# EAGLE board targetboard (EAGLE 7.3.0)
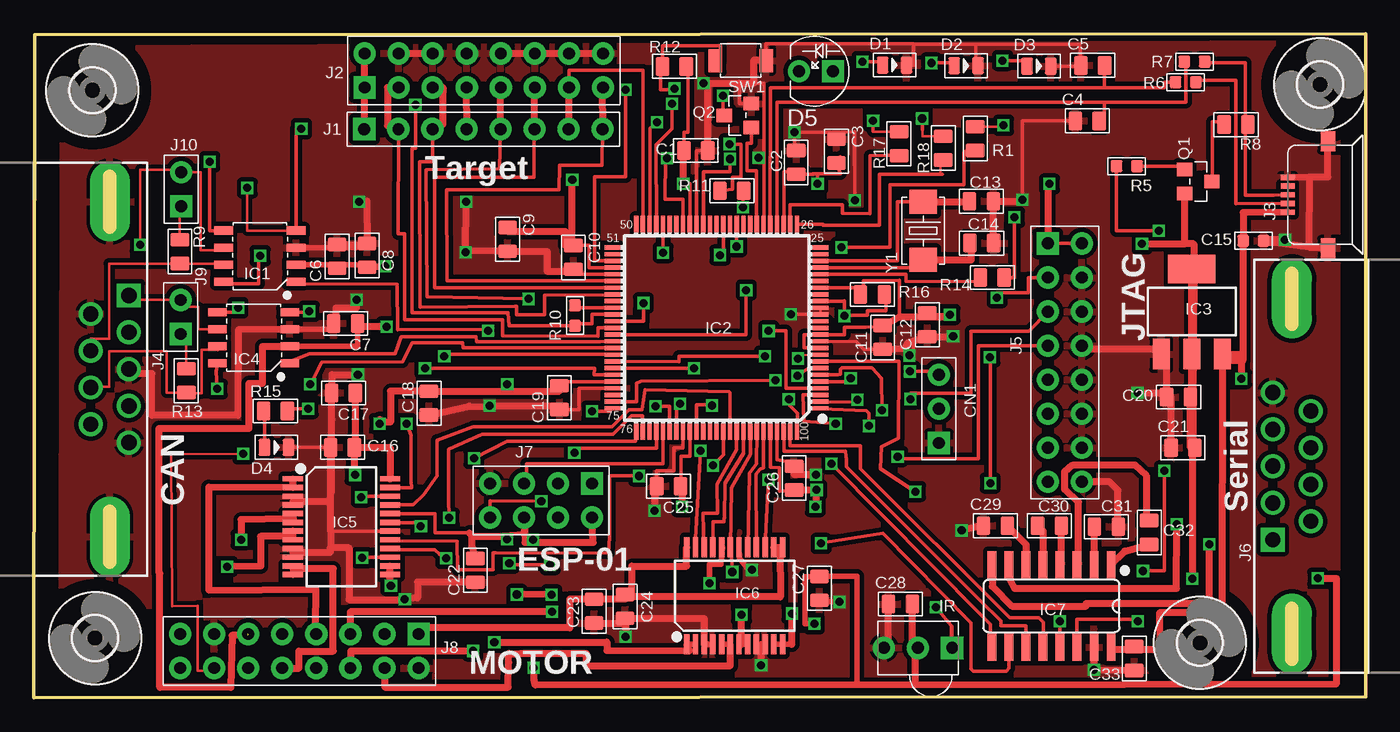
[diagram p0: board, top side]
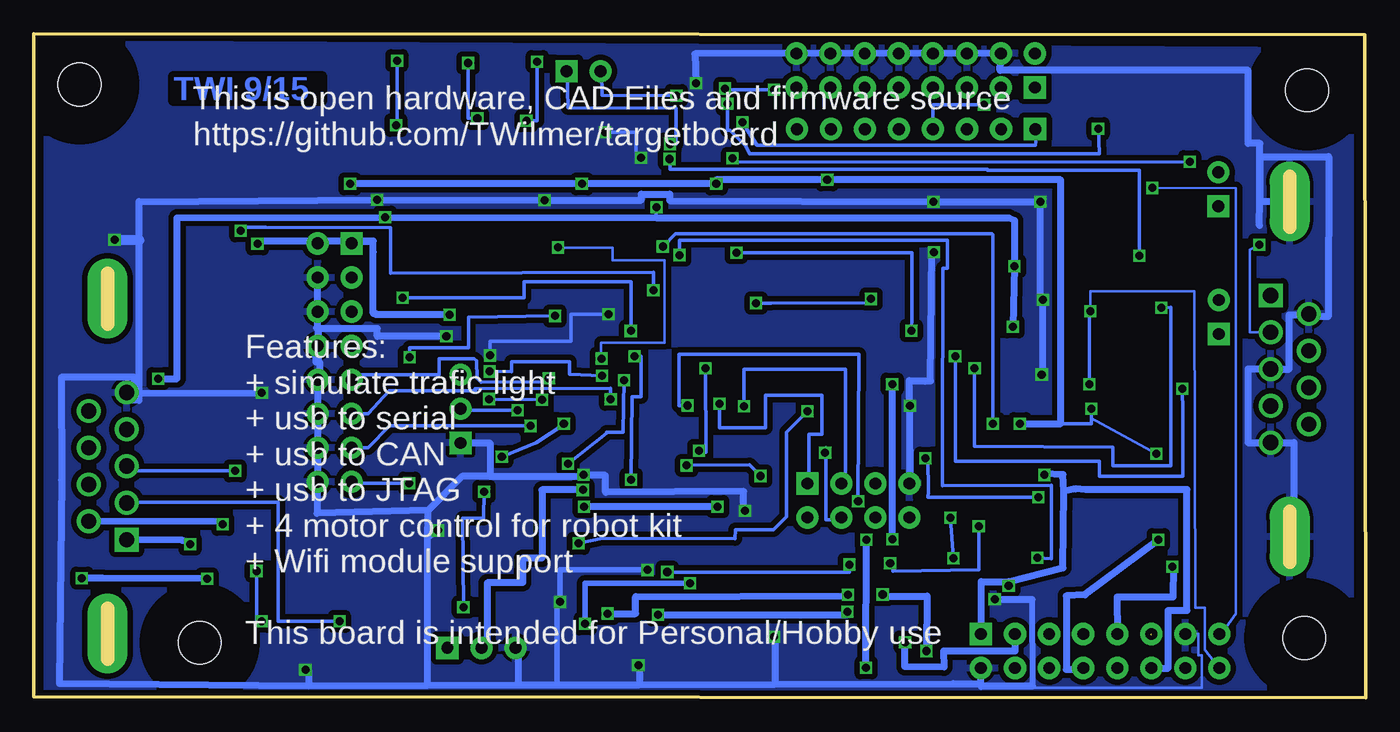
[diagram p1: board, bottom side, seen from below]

Size 99.44 x 49.57 mm. Coordinates in mm from the lower left corner, seen from the top.
Outline: 0,0 99.44,0.08 99.44,49.57 0.1,49.47 0,0
Copper layers (1*16): Top 0.035mm / dielectric 1.5mm / Bottom 0.035mm
Design rules "SeeedStudio_2layer_DRU_no_angle_20140221": minimum track width 7mil, minimum drill 12mil, track to track 7mil, track to pad 7mil, pad to pad 7mil, via to via 7mil, smd to smd 0mil, copper to edge 10mil, drill to drill 10mil, minimum pad ring 10mil, minimum via ring 6mil, stop-mask expansion 2mil, vias tented up to drill 100mil, thermal gap 10mil

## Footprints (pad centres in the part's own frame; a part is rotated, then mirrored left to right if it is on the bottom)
C0805 = smd 1.397 x 1.016: 1 0,0.889; 2 0,-0.889
C0603 = smd 0.889 x 0.889: 1 0,0.762; 2 0,-0.762
H3-2.54 = drill 0.889 pad 1.651 square: 1 0,2.54 | drill 0.889 pad 1.651: 2 0,0; 3 0,-2.54
LED-0805 = smd 0.889 x 1.27: + -0.889,0; - 0.889,0
LED2-2.54-D5.0MM = drill 0.889 pad 1.651 square: + -1.27,0 | drill 0.889 pad 1.651: - 1.27,0
3,2 = hole 3.2: 0,0
SOIC8-1.27-5X4MM = smd 0.6 x 1.4: 1 -1.905,-2.7; 2 -0.635,-2.7; 3 0.635,-2.7; 4 1.905,-2.7; 5 1.905,2.7; 6 0.635,2.7; 7 -0.635,2.7; 8 -1.905,2.7
LQFP100-0.5-13.8X13.8MM = smd 1.2 x 0.32: 1 -7.75,6; 2 -7.75,5.5; 3 -7.75,5; 4 -7.75,4.5; 5 -7.75,4; 6 -7.75,3.5; 7 -7.75,3; 8 -7.75,2.5; 9 -7.75,2; 10 -7.75,1.5; 11 -7.75,1; 12 -7.75,0.5; 13 -7.75,0; 14 -7.75,-0.5; 15 -7.75,-1; 16 -7.75,-1.5; 17 -7.75,-2; 18 -7.75,-2.5; 19 -7.75,-3; 20 -7.75,-3.5; 21 -7.75,-4; 22 -7.75,-4.5; 23 -7.75,-5; 24 -7.75,-5.5; 25 -7.75,-6; 51 7.75,-6; 52 7.75,-5.5; 53 7.75,-5; 54 7.75,-4.5; 55 7.75,-4; 56 7.75,-3.5; 57 7.75,-3; 58 7.75,-2.5; 59 7.75,-2; 60 7.75,-1.5; 61 7.75,-1; 62 7.75,-0.5; 63 7.75,0; 64 7.75,0.5; 65 7.75,1; 66 7.75,1.5; 67 7.75,2; 68 7.75,2.5; 69 7.75,3; 70 7.75,3.5; 71 7.75,4; 72 7.75,4.5; 73 7.75,5; 74 7.75,5.5; 75 7.75,6 | smd 0.32 x 1.2: 26 -6,-7.75; 27 -5.5,-7.75; 28 -5,-7.75; 29 -4.5,-7.75; 30 -4,-7.75; 31 -3.5,-7.75; 32 -3,-7.75; 33 -2.5,-7.75; 34 -2,-7.75; 35 -1.5,-7.75; 36 -1,-7.75; 37 -0.5,-7.75; 38 0,-7.75; 39 0.5,-7.75; 40 1,-7.75; 41 1.5,-7.75; 42 2,-7.75; 43 2.5,-7.75; 44 3,-7.75; 45 3.5,-7.75; 46 4,-7.75; 47 4.5,-7.75; 48 5,-7.75; 49 5.5,-7.75; 50 6,-7.75; 76 6,7.75; 77 5.5,7.75; 78 5,7.75; 79 4.5,7.75; 80 4,7.75; 81 3.5,7.75; 82 3,7.75; 83 2.5,7.75; 84 2,7.75; 85 1.5,7.75; 86 1,7.75; 87 0.5,7.75; 88 0,7.75; 89 -0.5,7.75; 90 -1,7.75; 91 -1.5,7.75; 92 -2,7.75; 93 -2.5,7.75; 94 -3,7.75; 95 -3.5,7.75; 96 -4,7.75; 97 -4.5,7.75; 98 -5,7.75; 99 -5.5,7.75; 100 -6,7.75
SOT-223 = smd 1.27 x 2.286: 1 -2.286,-3.175; 2 0,-3.175; 3 2.286,-3.175 | smd 3.556 x 2.159: TER 0,3.175
SSOP24-0.65-8.9X5.3MM = smd 0.4 x 1.5: 1 -3.575,-3.625; 2 -2.925,-3.625; 3 -2.275,-3.625; 4 -1.625,-3.625; 5 -0.975,-3.625; 6 -0.325,-3.625; 7 0.325,-3.625; 8 0.975,-3.625; 9 1.625,-3.625; 10 2.275,-3.625; 11 2.925,-3.625; 12 3.575,-3.625; 13 3.575,3.625; 14 2.925,3.625; 15 2.275,3.625; 16 1.625,3.625; 17 0.975,3.625; 18 0.325,3.625; 19 -0.325,3.625; 20 -0.975,3.625; 21 -1.625,3.625; 22 -2.275,3.625; 23 -2.925,3.625; 24 -3.575,3.625
SOIC16-1.27-10X3.9MM = smd 0.66 x 2.032: 1 -4.445,-3.073; 2 -3.175,-3.073; 3 -1.905,-3.073; 4 -0.635,-3.073; 5 0.635,-3.073; 6 1.905,-3.073; 7 3.175,-3.073; 8 4.445,-3.073; 9 4.445,3.073; 10 3.175,3.073; 11 1.905,3.073; 12 0.635,3.073; 13 -0.635,3.073; 14 -1.905,3.073; 15 -3.175,3.073; 16 -4.445,3.073
SNR3-2.54-6.95X6.0X5.6MM = drill 0.889 pad 1.651 square: 1 0,2.54 | drill 0.889 pad 1.651: 2 0,0; 3 0,-2.54
H8-2.54 = drill 0.889 pad 1.651 square: 1 0,8.89 | drill 0.889 pad 1.651: 2 0,6.35; 3 0,3.81; 4 0,1.27; 5 0,-1.27; 6 0,-3.81; 7 0,-6.35; 8 0,-8.89
H2X8-2.54 = drill 0.889 pad 1.651 square: 1 -1.27,8.89 | drill 0.889 pad 1.651: 2 -1.27,6.35; 3 -1.27,3.81; 4 -1.27,1.27; 5 -1.27,-1.27; 6 -1.27,-3.81; 7 -1.27,-6.35; 8 -1.27,-8.89; 9 1.27,-8.89; 10 1.27,-6.35; 11 1.27,-3.81; 12 1.27,-1.27; 13 1.27,1.27; 14 1.27,3.81; 15 1.27,6.35; 16 1.27,8.89
MICRO-USB5+2P-SMD-0.65 = smd 0.4 x 1.05: 1 -1.3,0; 2 -0.65,0; 3 0,0; 4 0.65,0; 5 1.3,0 | smd 1.5 x 1.1: 6 4,-3; 7 -4,-3
DSUB9+2P-2.77-90D-MALE = drill 1.143 pad 1.778 square: 1 -5.486,1.422 | drill 1.143 pad 1.778: 2 -2.743,1.422; 3 0,1.422; 4 2.743,1.422; 5 5.486,1.422; 6 -4.115,-1.422; 7 -1.372,-1.422; 8 1.372,-1.422; 9 4.115,-1.422 | drill 1 pad 3 long: G1 12.497,0; G2 -12.497,0
H2X4-2.54 = drill 0.889 pad 1.651 square: 1 -1.27,3.81 | drill 0.889 pad 1.651: 2 -1.27,1.27; 3 -1.27,-1.27; 4 -1.27,-3.81; 5 1.27,-3.81; 6 1.27,-1.27; 7 1.27,1.27; 8 1.27,3.81
H2-2.54 = drill 0.889 pad 1.651 square: 1 0,1.27 | drill 0.889 pad 1.651: 2 0,-1.27
SOT-23 = smd 1.016 x 1.143: 1 -0.889,-1.016; 2 0.889,-1.016; 3 0,1.016
R0805 = smd 1.397 x 1.016: 1 0,0.889; 2 0,-0.889
R0603 = smd 0.889 x 0.889: 1 0,0.762; 2 0,-0.762
SW2-2.6-3.0X2.5X1.2+0.4MM = smd 1 x 1.7: 1 -1.9,0; 2 1.9,0
X2-SMD-5.0X3.2X1.3MM = smd 1.778 x 2.032: 1 -2.159,0; 2 2.159,0

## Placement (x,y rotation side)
C1  100nf  [C0805]  49.43,40.84 270 top
C2  100nf  [C0805]  56.92,39.95 0 top
C3  10uf  [C0805]  59.92,40.79 0 top
C4  18pf  [C0805]  78.64,43.05 90 top
C5  18pf  [C0805]  79.04,47.19 90 top
C6  1uf  [C0805]  22.66,32.94 180 top
C7  100nf  [C0805]  23.29,27.94 270 top
C8  100nf  [C0805]  24.89,33.02 180 top
C9  100nf  [C0805]  35.38,34.21 0 top
C10  100nf  [C0805]  40.28,32.87 0 top
C11  100nf  [C0805]  63.37,26.9 180 top
C12  100nf  [C0805]  66.7,27.84 180 top
C13  18pf  [C0805]  70.74,37.06 270 top
C14  18pf  [C0805]  70.76,33.93 270 top
C15  10uf  [C0603]  91.03,34.11 270 top
C16  10uf  [C0805]  23.06,18.69 90 top
C17  100nf  [C0805]  23.14,22.76 270 top
C18  10uf  [C0805]  29.51,22 180 top
C19  100nf  [C0805]  39.24,22.4 180 top
C20  100nf  [C0805]  85.45,22.45 90 top
C21  10uf  [C0805]  85.78,18.67 90 top
C22  100nf  [C0805]  32.97,9.53 180 top
C23  100nf  [C0805]  41.83,6.48 0 top
C24  10uf  [C0805]  44.15,6.83 180 top
C25  100nf  [C0805]  47.4,15.8 270 top
C26  100nf  [C0805]  56.77,16.41 180 top
C27  100nf  [C0805]  58.65,8.18 180 top
C28  10uf  [C0805]  64.69,7.01 90 top
C29  1uf  [C0805]  71.78,12.85 90 top
C30  1uf  [C0805]  75.82,12.85 90 top
C31  1uf  [C0805]  80.06,12.78 90 top
C32  1uf  [C0805]  83.26,12.34 180 top
C33  100nf  [C0805]  82.14,2.95 180 top
CN1  DIP-BLACK-MALE-HEADER-VERT(3P-2.54)  [H3-2.54]  67.56,21.56 180 top
D1  SMD-LED-CLEAR-GREEN(0805)  [LED-0805]  64.26,47.22 0 top
D2  SMD-LED-CLEAR-YELLOW(0805)  [LED-0805]  69.6,47.17 0 top
D3  SMD-LED-CLEAR-RED(0805)  [LED-0805]  75.03,47.14 0 top
D4  SMD-LED-CLEAR-RED(0805)  [LED-0805]  18.14,18.69 0 top
D5  IR 940NM  [LED2-2.54-D5.0MM]  58.39,46.76 180 top
H1  MOUNT-HOLE3.2  [3,2]  4.39,45.34 0 top
H2  MOUNT-HOLE3.2  [3,2]  96.01,45.77 0 top
H3  MOUNT-HOLE3.2  [3,2]  4.6,4.47 0 top
H4  MOUNT-HOLE3.2  [3,2]  87.05,4.11 0 top
IC1  MCP2551  [SOIC8-1.27-5X4MM]  16.89,32.97 90 top
IC2  LPC1768 or LPC1768  [LQFP100-0.5-13.8X13.8MM]  50.98,27.61 180 top
IC3  PMIC-CJT1117-3.3(SOT223)  [SOT-223]  86.44,28.83 0 top
IC4  MCP2551  [SOIC8-1.27-5X4MM]  16.43,26.87 90 top
IC5  TB6612FNG  [SSOP24-0.65-8.9X5.3MM]  22.99,12.78 270 top
IC6  TB6612FNG  [SSOP24-0.65-8.9X5.3MM]  52.32,7.62 0 top
IC7  MAX232D  [SOIC16-1.27-10X3.9MM]  75.97,6.86 180 top
IR  TSOP2238  [SNR3-2.54-6.95X6.0X5.6MM]  66.01,3.73 270 top
J1  DIP-BLACK-MALE-HEADER-VERT(8P-2.54)  [H8-2.54]  33.58,42.44 90 top
J2  2x8p-2.54  [H2X8-2.54]  33.6,46.81 90 top
J3  USB  [MICRO-USB5+2P-SMD-0.65]  93.6,37.54 90 top
J4  CAN  [DSUB9+2P-2.77-90D-MALE]  5.69,24.54 270 top
J5  2x8p-2.54  [H2X8-2.54]  76.96,25.02 0 top
J6  Serial  [DSUB9+2P-2.77-90D-MALE]  93.9,17.3 90 top
J7  2X4P-2.54  [H2X4-2.54]  37.87,14.73 270 top
J8  2x8p-2.54  [H2X8-2.54]  19.84,3.51 270 top
J9  CAN2  [H2-2.54]  10.97,28.42 180 top
J10  CAN1  [H2-2.54]  11.02,37.95 180 top
Q1  PNP-24V  [SOT-23]  86.92,38.53 270 top
Q2  NMOSFET  [SOT-23]  52.55,43.46 90 top
R1  390R  [R0805]  70.28,41.73 180 top
R5  51R  [R0603]  81.58,39.67 90 top
R6  33.2R  [R0603]  85.98,45.95 90 top
R7  33.2R  [R0603]  86.64,47.47 90 top
R8  1.5K  [R0805]  89.74,42.77 270 top
R9  120R  [R0805]  10.92,33.3 0 top
R10  330R  [R0603]  40.41,28.52 0 top
R11  100R  [R0805]  52.12,37.85 90 top
R12  1.5K  [R0805]  47.83,47.12 90 top
R13  120R  [R0805]  11.4,23.67 0 top
R14  1.5K  [R0805]  71.55,31.37 270 top
R15  100R  [R0805]  18.06,21.41 90 top
R16  2K  [R0805]  62.61,30.1 270 top
R17  390R  [R0805]  64.59,41.35 180 top
R18  390R  [R0805]  67.89,41.02 180 top
SW1  SW  [SW2-2.6-3.0X2.5X1.2+0.4MM]  52.78,47.55 180 top
Y1  12MHZ  [X2-SMD-5.0X3.2X1.3MM]  66.4,34.85 90 top

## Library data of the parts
C1 C2 C7-C12 C17 C19 C20 C22 C23 C25-C27 C33 = Seeed-OPL-Capacitor; MPN: CC0805KRX7R9BB104
C3 C16 C18 C21 C24 C28 = Seeed-OPL-Capacitor; MPN: CC0805KKX5R8BB106
C4 C5 C13 C14 = Seeed-OPL-Capacitor
C6 C29-C32 = Seeed-OPL-Capacitor; MPN: CC0805KKX7R8BB105
C15 = Seeed-OPL-Capacitor; MPN: CC0603KRX5R6BB106
CN1 J4 J6 J7 = Seeed-OPL-Connector
D1 = Seeed-OPL-Diode; MPN: 17-215SYGC/S530-E2/TR8
D2 = Seeed-OPL-Diode; MPN: 17-215UYC/S530-A3/TR8
D3 D4 = Seeed-OPL-Diode; MPN: 17-215SURC/S530-A2/TR8
D5 = Seeed-OPL-Diode; MPN: IR523B-W60W1
H1-H4 = holes
IC1 IC4 = Seeed-OPL-ic; MPN: MCP2551-I/SN
IC2 = Seeed-OPL-ic; MPN: LPC1768FBD100
IC3 = Seeed-OPL-ic; MPN: CJT1117-3.3
IC5 IC6 = Seeed-OPL-ic; MPN: TB6612FNG-O/C8/EL
IC7 = Seeed-OPL-ic; MPN: MAX232D
IR = Seeed-OPL-sensor
J1 = Seeed-OPL-Connector; MPN: P125-1108A1BS116A1
J2 J5 J8 = Seeed-OPL-Connector; MPN: P125-1216A0AS116A1
J3 = Seeed-OPL-Connector; MPN: ST-USB-001L
J9 J10 = Seeed-OPL-Connector; MPN: P125-1102A0BS116A3
Q1 = Seeed-OPL-Transistor; MPN: S8550
Q2 = Seeed-OPL-Transistor; MPN: 2N7002,215
R1 R17 R18 = Seeed-OPL-Resistor; MPN: RC0805JR-07390RL
R5 = Seeed-OPL-Resistor; MPN: RC0603FR-0751RL
R6 R7 = Seeed-OPL-Resistor; MPN: RC0603FR-0733R2L
R8 R12 R14 = Seeed-OPL-Resistor; MPN: RC0805FR-071K5L
R9 R13 = Seeed-OPL-Resistor; MPN: RC0805JR-07120RL
R10 = Seeed-OPL-Resistor; MPN: RC0603FR-07330RL
R11 R15 = Seeed-OPL-Resistor; MPN: RC0805JR-07100RL
R16 = Seeed-OPL-Resistor; MPN: RC0805JR-072KL
SW1 = Seeed-OPL-Switch
Y1 = Seeed-OPL-crystal-osctllator; MPN: 5032/2P

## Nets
+12V: C16.2 C17.1 C23.1 C24.2 IC5.13 IC5.14 IC5.24 IC6.13 IC6.14 IC6.24 J8.1 J8.11
CAN1_H: IC1.7 J4.7 R9.2
CAN1_L: IC1.6 J4.2 J10.2
CAN1_REF: IC1.5 IC2.43
CAN1_RS: IC1.8 IC2.40
CAN1_RX: IC1.4 IC2.47 J8.8
CAN1_TX: IC1.1 IC2.46
CAN2_H: IC4.7 J4.8 R13.2
CAN2_L: IC4.6 J4.1 J9.2
CAN2_REF: IC2.70 IC4.5
CAN2_RS: IC2.67 IC4.8
CAN2_RX: IC2.66 IC4.4 J8.9
CAN2_TX: IC2.65 IC4.1
CM1A: IC2.91 IC6.22
CM1B: IC2.92 IC6.21
CM2A: IC2.94 IC6.17
CM2B: IC2.95 IC6.16
CM3A: IC2.76 IC5.22
CM3B: IC2.90 IC5.21
CM4A: IC2.89 IC5.17
CM4B: IC2.77 IC5.16
DM: J3.2 R6.2
DP: J3.3 R7.2 R8.1
EDM: C5.2 IC2.30 R6.1
EDP: C4.2 IC2.29 R7.1
ESP_0: IC2.81 J7.2
ESP_2: IC2.80 J7.3
ESP_RST: IC2.79 J7.7
GND: C1.1 C2.1 C3.1 C4.1 C5.1 C6.2 C7.2 C8.2 C9.2 C10.2 C11.1 C12.1 C13.1 C14.1 C15.1 C16.1 C17.2 C18.1 C19.1 C20.1 C21.1 C22.1 C23.2 C24.1 C25.2 C26.2 C27.1 C28.1 C29.1 C31.2 C33.1 CN1.1 D1.- D2.- D3.- D4.- IC1.3 IC2.11 IC2.15 IC2.16 IC2.31 IC2.41 IC2.55 IC2.72 IC2.83 IC2.97 IC3.1 IC4.3 IC5.3 IC5.4 IC5.9 IC5.10 IC5.18 IC6.3 IC6.4 IC6.9 IC6.10 IC6.18 IC7.15 IR.3 J2.9 J2.10 J2.11 J2.12 J2.13 J2.14 J2.15 J3.5 J3.6 J3.7 J4.3 J4.5 J4.6 J4.G1 J4.G2 J5.9 J5.10 J5.11 J5.12 J5.13 J5.14 J5.15 J6.5 J7.4 J8.7 J8.16 Q2.2 SW1.1
IR_IN: IC2.8 IR.1
IR_SEND: IC2.32 Q2.1
LED1: IC2.9 R1.1
LED2: IC2.27 R17.1
LED3: IC2.26 R18.1
M1A: IC6.1 IC6.2 J8.2
M1B: IC6.5 IC6.6 J8.15
M2A: IC6.7 IC6.8 J8.3
M2B: IC6.11 IC6.12 J8.14
M3A: IC5.1 IC5.2 J8.4
M3B: IC5.5 IC5.6 J8.13
M4A: IC5.7 IC5.8 J8.5
M4B: IC5.11 IC5.12 J8.12
N$1: IC2.48 J1.1 J2.1 J2.16
N$2: IC2.53 R12.1 SW1.2
N$3: D2.+ R18.2
N$4: D1.+ R17.2
N$5: D3.+ R1.2
N$6: C14.2 IC2.22 Y1.1
N$7: Q1.3 R8.2
N$8: C13.2 IC2.23 Y1.2
N$9: Q1.1 R5.2
N$10: IC2.21 R14.2
N$11: J10.1 R9.1
N$13: J9.1 R13.1
N$14: D5.+ R11.1
N$15: C30.2 IC7.4
N$16: C30.1 IC7.5
N$17: C32.1 IC7.1
N$18: C32.2 IC7.3
N$19: C29.2 IC7.6
N$20: C31.1 IC7.2
N$21: D5.- Q2.3
N$22: IC2.60 R10.1
N$24: D4.+ R15.1
NTRST: IC2.4 J5.2
P2_9: IC2.64 R5.1
PWM1: IC2.69 IC6.23
PWM2: IC2.68 IC6.15
PWM3: IC2.35 IC5.23
PWM4: IC2.37 IC5.15
RST: IC2.17 J5.8 R16.1
RTCK: IC2.100 J5.6
RX3: CN1.2 IC2.6
RX_TO_TX: IC2.85 J7.5
RXD0: IC2.99 IC7.12
RXD1: IC2.74 IC7.9
SER1_RX: IC7.13 J6.2
SER1_TX: IC7.14 J6.3
SER2_RX: IC7.8 J6.1
SER2_TX: IC7.7 J6.6
STBY: IC2.93 IC5.19 IC6.19
T_RTCK: IC2.57 J1.6 J2.6
T_SRST: IC2.56 J1.8 J2.8
T_SWDCLK: IC2.62 J1.5 J2.5
T_SWDIO: IC2.61 J1.4 J2.4 R10.2
T_SWO: IC2.49 J1.7 J2.7
T_TDI: IC2.58 J1.3 J2.3
T_TRST: IC2.63 J1.2 J2.2
TCK: IC2.5 J5.5
TDI: IC2.2 J5.3
TDO: IC2.1 J5.7
TMS: IC2.3 J5.4
TX3: CN1.3 IC2.7
TX_TO_RX: IC2.82 J7.1
TXD0: IC2.98 IC7.11
TXD1: IC2.75 IC7.10
VCC: C6.1 C7.1 C8.1 C15.2 C33.2 IC1.2 IC3.3 IC4.2 IC7.16 J3.1 J8.6 R11.2 R14.1
VDD: C1.2 C2.2 C3.2 C9.1 C10.1 C11.2 C12.2 C18.2 C19.2 C20.2 C21.2 C22.2 C25.1 C26.1 C27.2 C28.2 IC2.10 IC2.12 IC2.19 IC2.28 IC2.42 IC2.54 IC2.71 IC2.84 IC2.96 IC3.2 IC3.TER IC5.20 IC6.20 IR.2 J5.1 J5.16 J7.6 J7.8 J8.10 Q1.2 R12.2 R15.2 R16.2

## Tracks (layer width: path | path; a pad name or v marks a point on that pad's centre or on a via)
+12V  (via drill 0.6)
  Top 0.178: IC6.13 55.91,11.25 55.7,11.24
  Top 0.406: C23.1 40.56,7.37 40.56,7.39
  Top 0.508: 24,22.76 C17.1 24.03,18.69 | 24.03,18.69 C16.2 23.95,16.64 v24,16.64 | C24.2 44.15,7.39 40.56,7.39 40.03,7.39 40.03,5.23 28.73,5.23 J8.1 | C24.2 44.65,7.72 44.65,9.83 48.75,9.83 IC6.24 | IC6.14 55.7,11.24 55.73,7.54 44.17,7.54 C24.2 | 24.03,18.69 26.61,18.69 IC5.24 | IC5.13 IC5.14 26.61,8.38 v26.67,8.38
  Bottom 0.508: 26.67,8.69 22.61,9.7 22.53,15.42 | 22.53,15.42 22.61,16.66 24,16.74 v24,16.64 | 26.67,8.69 28.73,8.69 J8.1 | 26.67,8.69 v26.67,8.38 | J8.11 14.76,2.23 14.76,6.53 13.36,6.53 13.36,15.54 20.93,15.54 21.67,15.6 22.53,15.42
CAN1_H
  Top 0.178: IC1.7 14.19,32.41 R9.2 5.64,32.41 5.64,26.8 4.27,26.8 J4.7
CAN1_L  (via drill 0.6)
  Top 0.178: v7.95,33.81 7.98,39.42 11.02,39.4 J10.2 12.47,39.22 12.47,33.4 14.19,33.4
  Top 0.254: 14.19,33.4 IC1.6
  Bottom 0.178: J4.2 8.66,27.28 8.66,33.43 v7.95,33.81
CAN1_REF  (via drill 0.6)
  Top 0.254: IC1.5 13.16,34.87 v13.16,40 | v47.27,40.26 47.17,40.28 47.14,37.21 48.45,37.21 IC2.43
  Bottom 0.254: v13.16,40 47.17,39.98 v47.27,40.26
CAN1_RS  (via drill 0.6)
  Top 0.254: IC2.40 49.99,39.27 51.97,39.27 v51.97,40.21 | v16.92,32.99 16.82,32.99 16.82,30.89 14.19,30.89 IC1.8
  Bottom 0.254: v51.97,40.21 51.94,40.21 51.94,39.45 28.27,39.45 28.27,39.37 16.92,39.37 v16.92,32.99
CAN1_RX  (via drill 0.6)
  Top 0.178: IC1.4 15.95,34.87 v15.95,38.05
  Top 0.254: IC2.47 46.51,35.36 46.46,41.27 47.65,42.47 v47.65,44.32 | v19.99,42.47 19.59,42.47 IC1.4
  Bottom 0.178: v15.95,38.05 9.73,38.02 9.73,29.16 9.7,29.16 9.7,6.27 10.47,5.23 10.59,4.67
  Bottom 0.254: v47.65,44.32 47.65,42.37 47.47,42.37 46.36,41.25 46.3,41.25 46,40.61 19.91,40.61 v19.99,42.47
  Bottom 0.508: 10.59,4.67 10.95,4.67 J8.8
CAN1_TX  (via drill 0.6)
  Top 0.254: IC2.46 v46.99,33.22 | v33.93,27.41 33.88,27.61 33.93,27.51 27.18,27.48 27.13,30.86 19.59,30.89 IC1.1
  Bottom 0.254: v46.99,33.22 33.88,33.22 33.88,28.02 33.93,27.81 v33.93,27.41
CAN2_H
  Top 0.178: 13.73,25.98 12.55,25.98 12.55,22.73 11.4,22.73 R13.2 9.93,22.78 9.93,25.88 5.64,25.88 5.64,23.22 4.27,23.22 J4.8
  Top 0.254: 13.73,25.98 IC4.7
CAN2_L
  Top 0.178: IC4.6 12.29,27.51 12.29,29.18 10.97,29.18 J9.2 7.11,29.69 J4.1
CAN2_REF  (via drill 0.6)
  Top 0.254: IC4.5 15.27,28.78 v15.27,29.11 | v29.21,24.61 41.86,24.61 41.83,24.13 43.2,24.13 IC2.70
  Bottom 0.254: v15.27,29.11 14.55,29.13 14.55,18.8 14.58,18.8 14.58,17.32 18.9,17.32 18.9,18.72 29.24,18.8 v29.21,24.61
CAN2_RS  (via drill 0.6)
  Top 0.254: IC4.8 13.64,24.36 v13.72,23.06 | v30.66,25.5 31.01,25.76 31.01,25.63 43.23,25.63 IC2.67
  Bottom 0.254: v13.72,23.06 13.67,21.31 13.67,16.54 19.89,16.54 19.89,17.68 30.66,17.65 v30.66,25.5
CAN2_RX  (via drill 0.6)
  Top 0.254: IC4.4 20.57,28.78 v20.57,28.85 | v20.65,23.39 20.68,23.39 21.51,25.04 27.56,25.07 28.27,26.52 32,26.52 32.06,26.11 43.28,26.11 IC2.66
  Bottom 0.178: J8.9 12.04,3.61 12.04,6.73 12.75,6.73 12.8,30.35 20.57,30.35 v20.57,28.85
  Bottom 0.254: v20.57,28.85 20.65,28.85 v20.65,23.39
CAN2_TX
  Top 0.254: IC4.1 18.52,24.87 20.6,25.68 26.98,25.68 27.43,26.95 33.02,26.95 33.07,26.57 42.29,26.57 IC2.65
CM1A
  Top 0.254: IC6.22 49.97,13.78 51.05,13.77 51,15.95 52.45,18.52 52.48,19.78 IC2.91
CM1B
  Top 0.254: IC6.21 50.7,13.13 51.54,13.13 51.54,13.41 51.56,13.41 51.61,16.03 52.98,18.26 52.98,19.69 IC2.92
CM2A
  Top 0.254: IC6.17 53.31,11.24 53.42,16.76 53.95,17.47 IC2.94
CM2B
  Top 0.254: IC2.95 54.48,17.19 54.23,17.07 53.92,16.69 IC6.16
CM3A  (via drill 0.6)
  Top 0.254: IC5.22 24.46,15.05 v24.46,14.99 | v32.87,17.88 35.36,19.15 44.93,19.15 44.93,19.58 IC2.76
  Bottom 0.254: v24.46,14.99 32.69,14.96 32.66,15.39 32.69,17.88 32.61,17.96 v32.87,17.88
CM3B
  Top 0.254: IC2.90 51.98,22.77 51.92,22.83 45.62,22.99 45.42,21.51 44.45,21.51 43.18,20.24 32.82,20.24 30.12,19.23 30.12,16.59 29.11,15.16 28.35,14.4 IC5.21
CM4A  (via drill 0.6)
  Top 0.254: IC2.89 51.48,18.15 v50.7,17.35 | v45.19,16.56 42.98,16.56 42.98,12.04 42.93,10.79 34.49,10.85 34.29,10.85 34.29,9.55 31.65,9.55 31.65,9.58 31.62,11.68 26.59,11.73 IC5.17
  Bottom 0.254: v50.7,17.35 46.03,17.4 v45.19,16.56
CM4B  (via drill 0.6)
  Top 0.254: IC2.77 45.47,19.86 45.47,21.06 44.63,21.06 43.23,19.66 33.48,19.66 30.96,18.57 30.96,14.93 v31.01,13.44 | v30.79,10.41 30.25,10.77 29.95,11.07 26.66,11.07 26.66,11.1 IC5.16
  Bottom 0.254: v31.01,13.44 v30.79,10.41
DM
  Top 0.254: J3.2 89.74,36.87 89.74,46.08 86.69,46.08 R6.2
DP
  Top 0.254: J3.3 92.56,37.52 90.45,37.52 90.45,42.77 | 90.45,42.77 90.45,47.4 87.4,47.4 R7.2 | R8.1 90.45,42.77
EDM
  Top 0.254: 79.93,45.54 79.93,45.52 55,45.52 IC2.30 | R6.1 84.4,45.95 84.4,45.54 79.93,45.54 | 79.93,45.54 C5.2
EDP
  Top 0.254: R7.1 85.98,47.47 85.98,44.45 79.93,44.45 | 79.93,44.45 55.48,44.45 IC2.29 | C4.2 79.93,43.05 79.93,44.45
ESP_0  (via drill 0.6)
  Top 0.254: v46.41,21.77 47.48,21.77 IC2.81
  Bottom 0.254: J7.2 38.86,16 38.86,24.54 46.41,24.54 v46.41,21.77
ESP_2
  Top 0.254: J7.3 36.8,16 36.8,17.47 46.98,17.47 IC2.80
ESP_RST  (via drill 0.6)
  Top 0.254: IC2.79 46.48,18.64 40.36,18.64 v40.36,18.29
  Bottom 0.254: v40.36,18.29 40.31,18.67 40.31,13.28 39.14,13.28 J7.7
GND  (via drill 0.6)
  Top 0.178: 34.01,21.74 33.81,21.74 33.81,21.77 v34.04,21.79 | IC2.16 IC2.15
  Top 0.254: 91.8,34.09 C15.1 | IC2.97 55.5,19.86 55.47,17.78 56.77,17.55 C26.2 | IC2.83 48.49,18.67 47.8,18.67 47.8,16.94 46.51,16.94 C25.2 | IC2.72 40.72,23.11 40.72,21.49 39.24,21.49 C19.1 | C1.1 49.48,40.84 IC2.41 | IC2.31 54.51,35.36 54.51,45.85 53.77,45.85 53.77,45.87 | 60.22,42.21 v56.79,42.21 56.79,40.84 C2.1 | 60.22,42.21 C3.1 | 60.22,42.21 61.27,42.24 v61.29,37.13 | D1.- 65.66,47.22 | SW1.1 54.68,48.79 65.68,48.79 65.71,47.22 65.66,47.22 | 65.66,47.22 65.66,48.77 70.33,48.77 | 70.33,48.77 78.11,48.77 C5.1 | C5.1 77.93,47.19 77.93,47.22 77.95,47.22 | D3.- 78.16,47.14 C5.1 | C4.1 73.79,43.05 v73.79,37.16 | D2.- 70.33,47.17 70.33,48.77 | IC2.11 61.42,26.59 61.93,26.03 62.84,26.03 63.65,26.06 63.45,26.25 C11.1 | IC2.15 v56.52,28.61 v56.52,28.63 | v65.38,25.55 65.66,25.55 65.66,26.64 | IC5.18 22.17,12.45 | 22.17,18.36 C16.1 D4.- | IC5.3 IC5.4 | IC5.10 IC5.9 | C10.2 40.61,31.98 40.61,31.6 43.23,31.6 IC2.55 | v54.1,40.31 54.41,40.28 54.41,40.26 | Q2.2 52.68,44.35 52.68,45.87
  Top 0.356: 19.36,14.66 IC5.4 | 19.36,10.85 IC5.9
  Top 0.406: IC4.3 22.4,27.51 C7.2 | IC1.3 24.05,33.6 C8.2 | IC6.3 IC6.4 | IC6.9 54.31,3.99 IC6.10 | 44.17,5.59 44.15,5.59 C24.1 | IC6.18 52.68,10.41 53.34,9.55 v53.62,9.55 | v60.15,7.16 58.62,7.16 C27.1
  Top 0.508: J3.5 95.2,38.87 | 95.2,38.87 95.17,33.63 | 95.17,33.63 91.8,34.09 | C20.1 84.56,25.65 IC3.1 83.79,26.01 77.8,26.01 | C20.1 84.89,22.45 C21.1 | v24.31,37.03 24.87,37.06 C8.2 24.05,33.81 C6.2 | C7.2 22.58,27.94 22.58,29.11 24.1,29.11 v24.1,29.72 | v32.28,37.03 v32.26,33.25 32.41,33.38 C9.2 38.33,33.32 38.33,31.83 40.28,31.83 C10.2 | IR.3 63.81,3.73 C28.1 | C28.1 63.63,7.01 | v50.01,45.87 50.32,45.87 | 50.32,45.87 C1.1 | 50.32,45.87 52.68,45.87 53.77,45.87 53.77,47.6 54.68,47.6 SW1.1 | C16.1 22.25,18.69 C17.2 | 22.25,20.78 C17.2 | C17.2 22.28,22.76 22.28,24.13 v24.21,24.13 | C18.1 32.52,21.77 33.81,21.74 | v34.04,21.79 39.24,21.79 C19.1 | C25.2 46.36,15.8 v46.36,13.97 | v58.39,16.66 56.77,16.66 C26.2 | C29.1 69.29,12.52 v69.27,12.5 | C11.1 65.02,26.09 65.23,26.49 65.66,26.64 66.62,26.9 C12.1 68.63,26.95 v68.63,26.97 | v73.79,37.16 73.79,37.06 C13.1 71.63,33.93 C14.1 | C28.1 63.6,7.01 | C24.1 50.05,5.94 IC6.3 | C23.2 44.17,5.59 v44.17,4.57 | 54.31,3.99 v54.31,2.44 | IC4.3 15.29,27.46 15.24,21.08 8.84,21.08 8.84,24.21 7.06,24.21 J4.3 | C31.2 80.92,12.8 80.92,15.49 80.29,16.13 J5.9 | C33.1 79.15,2.03 v79.15,2.11 IC7.15 | 19.36,14.66 22.15,14.66 22.15,15.27 22.2,15.27 22.2,18.36 22.17,18.36 22.17,12.45 22.17,11.2 | 22.17,11.2 22.17,11.15 22.12,11.15 22.12,10.85 19.36,10.85 | v82.4,22.76 84.56,22.76 C20.1 | C22.1 28.65,8.64 28.65,7.47 v27.71,7.37 | 22.17,11.2 23.55,11.2 23.55,7.34 27.43,7.34 27.43,7.42 | J2.15 J2.14 30.25,48.08 30.25,48.06 | J2.12 J2.11 J2.10 J2.9 | 95.2,38.87 96.6,38.87 J3.6 | 95.17,33.63 96.57,33.63 J3.7
  Top 0.737: C15.1 93.4,34.11 v93.4,34.19
  Bottom 0.178: IR.3 63.27,3.61 | J4.G1 5.69,12.6 5.46,12.6 5.39,12.7 | 24.89,0.89 24.87,0.76 12.24,0.76 12.24,3.2 12.5,3.2 12.5,4.8 12.6,4.8 J8.7
  Bottom 0.254: 4.27,28.57 J4.6 | v56.52,28.63 59.31,28.63 59.31,26.61 65.38,26.61 v65.38,25.55 | 65.38,16.69 67.46,16.54 | 78.28,13.77 78.23,13.82 | 97.44,15.93 97.34,16.25 | v56.79,42.21 54.48,42.21 54.48,40.33 53.95,40.33 v54.1,40.31
  Bottom 0.406: v53.62,9.55 60.15,9.55 v60.15,7.16 60.38,7.16 60.38,0.98
  Bottom 0.457: 24.92,7.37 24.89,0.89
  Bottom 0.508: 34.09,23.67 34.01,16.84 J7.4 34.04,16 v34.04,21.79 | 34.09,23.67 32.49,23.65 | 32.49,23.65 32.41,33.45 v32.26,33.25 | J6.5 92.53,22.83 92.53,22.94 92.61,22.94 92.61,23.01 91.77,23.01 91.77,23.6 91.9,23.6 91.9,23.93 97.36,23.93 97.34,16.25 97.51,1.09 78.92,0.92 | 78.92,0.92 70.05,0.95 | 70.05,0.95 63.27,0.97 | 63.27,0.97 60.38,0.98 54.23,1 | 54.23,1 44.12,1.03 | 44.12,1.03 30.81,1.07 28.73,1.07 J8.16 28.73,0.86 24.89,0.89 | v50.01,45.87 50.09,48.06 J2.15 27.31,46.81 8.79,46.81 8.79,41.38 7.93,41.38 7.93,37.36 | v24.21,24.13 24.1,24.13 v24.1,29.72 24.31,29.72 v24.31,37.03 v32.28,37.03 51.97,37.11 51.97,37.59 54.08,37.59 54.08,37.13 v61.29,37.13 v73.79,37.16 91.57,37.03 91.57,34.09 91.57,22.2 92.35,22.2 J6.5 | 34.09,23.67 32.92,23.64 32.49,23.65 | v46.36,13.97 46.46,13.97 46.46,15.42 56.74,15.34 56.77,16.61 58.42,16.61 v58.39,16.66 58.39,16.54 65.38,16.54 | CN1.1 65.38,19.02 65.38,16.69 65.38,16.54 | 65.38,16.54 67.46,16.54 | 67.46,16.54 70.03,13.94 70.05,11.61 | v69.27,12.5 70.05,11.96 70.05,11.61 | 70.05,11.61 70.05,0.95 | v68.63,26.97 73.79,26.97 73.79,27.56 78.16,27.56 | 78.16,27.56 78.31,27.56 78.31,27.66 78.23,27.66 J5.14 J5.15 | J5.13 78.38,26.29 78.38,25.07 78.16,25.07 | 78.16,25.07 78.16,27.56 | 78.16,25.07 78.11,25.07 78.11,23.11 78.23,23.11 J5.12 J5.11 J5.10 J5.9 78.23,13.82 | 63.6,3.61 63.27,3.61 63.27,0.97 | v44.17,4.57 44.12,4.57 44.12,1.03 | v54.31,2.44 54.23,2.44 54.23,1 | 5.39,12.7 5.39,19.05 J4.5 8.81,19.05 8.81,24.54 J4.3 5.74,24.54 5.74,28.57 4.27,28.57 | 7.95,35.25 7.93,37.12 | 7.93,37.12 7.93,37.36 | 67.46,16.54 70,14 78.28,13.77 | v79.15,2.11 78.92,2.11 78.92,0.92
  Bottom 0.508: J6.5 82.4,22.73 v82.4,22.76 | v27.71,7.37 24.92,7.37 | 7.93,37.36 7.9,37.36 7.87,40.39 2.79,40.39 2.82,28.45 4.27,28.45 J4.6 | J4.G2 7.93,37.03 7.93,37.12
  Bottom 0.737: v93.4,34.19 91.57,34.19 91.57,34.09
  pour Bottom (isolate 0.406): 1.17,0.3 98.42,0.3 98.42,48.84 1.17,48.31
  pour Top (isolate 0.33): 2.24,48.44 2.08,0.2 97.28,0.2 97.28,48.82
IR_IN  (via drill 0.6)
  Top 0.254: IC2.8 64.57,25.11 64.54,19.38 63.27,18.74 63.2,17.09 v65.81,15.39 | v67.36,6.78 68.5,5.38 68.48,3.91 68.55,5.33 IR.1
  Bottom 0.254: v65.81,15.39 65.86,13.41 67.41,13.41 v67.36,6.78
IR_SEND
  Top 0.254: IC2.32 53.95,35.36 53.95,39.34 53.26,39.34 53.26,41.4 53.57,41.4 Q2.1
LED1  (via drill 0.6)
  Top 0.178: IC2.9 57.28,25.58 v57.05,25.32 | R1.1 69.42,40.84 69.42,40.54
  Top 0.254: v60.3,33.61 63.91,33.61 63.91,38.3 69.42,38.3 69.42,40.54 69.42,40.74 70.82,40.74
  Bottom 0.178: v57.05,25.32 57.07,25.78 57.07,26.49 52.35,26.49 52.35,32.64 56.24,32.64 56.24,33.58 60.3,33.58 v60.3,33.61
LED2
  Top 0.178: R17.1 63.78,40.46 63.78,40.5
  Top 0.254: IC2.27 56.46,35.36 56.46,36.78 60.38,36.78 60.38,36.17 62.41,36.12 62.41,40.46 63.78,40.5 64.36,40.51
LED3
  Top 0.178: R18.1 67.67,40.13 67.67,39.06
  Top 0.254: IC2.26 58.93,35.36 58.93,35.28 63.14,35.28 63.14,39.06 67.67,39.06 67.82,39.06
M1A  (via drill 0.6)
  Top 0.406: IC6.1 IC6.2
  Top 0.508: v34.39,4.17 42.8,4.17 42.8,3.56 42.82,3.56 48.98,3.53 IC6.1
  Bottom 0.508: J8.2 26.19,3.5 31.52,3.5 31.5,2.31 34.42,2.34 v34.39,4.17
M1B
  Top 0.406: IC6.5 IC6.6
  Top 0.508: J8.15 26.24,2.23 26.21,0.81 35.43,0.81 35.46,2.64 35.46,3.3 36.35,3.3 36.35,3.33 41.25,3.33 41.25,2.41 | 41.25,2.41 41.3,2.39 | 41.25,2.41 52,2.41 IC6.6
M2A  (via drill 0.6)
  Top 0.406: IC6.8 52.83,3.99 IC6.7
  Top 0.508: 52.83,3.99 v52.83,6.2 | v38.71,6.43 23.65,6.43 J8.3
  Bottom 0.508: v52.83,6.2 38.71,6.2 v38.71,6.43
M2B  (via drill 0.6)
  Top 0.406: 56.59,3.99 IC6.12 IC6.11
  Top 0.508: 56.59,3.99 v56.59,6.3 | v38.66,7.7 v36.07,7.72 | v32.79,3.5 23.67,3.5 J8.14
  Bottom 0.508: v56.59,6.3 54.51,6.3 54.51,7.57 38.94,7.65 38.76,7.7 v38.66,7.7 | v36.07,7.72 36.14,7.85 35.97,7.85 36.14,7.59 32.77,7.59 v32.79,3.5
M3A
  Top 0.508: IC5.1 IC5.2 13.08,15.73 13.08,8.05 21.06,8.1 21.03,5.31 21.11,5.31 J8.4
M3B  (via drill 0.6)
  Top 0.254: IC5.6 19.38,13.1 19.38,13.36
  Top 0.356: IC5.6 IC5.5
  Top 0.508: 19.36,13.39 19.38,13.39 19.38,13.36 19.08,13.36 15.49,13.3 v15.49,11.81
  Bottom 0.508: v15.49,11.81 15.44,11.81 20.98,7.7 22.38,7.62 22.38,2.13 21.11,2.13 J8.13
M4A  (via drill 0.6)
  Top 0.254: IC5.8 IC5.7
  Top 0.508: IC5.7 19.33,12.06 16.94,12.06 | 16.94,12.06 16.97,11.99 | 16.94,12.06 16.97,9.83 14.4,9.8 v14.45,9.8
  Bottom 0.508: v14.45,9.8 14.38,9.83 14.4,7.52 18.59,7.52 J8.5
M4B
  Top 0.254: IC5.12 IC5.11
  Top 0.508: J8.12 19.81,2.23 19.81,3.5 22.38,3.5 22.38,9.65 19.36,9.65 IC5.12
N$1  (via drill 0.6)
  Top 0.254: IC2.48 46,35.36 46,42.52 46.48,42.85 v46.53,42.95
  Top 0.508: J1.1 24.71,42.85 J2.1 J2.16
  Bottom 0.254: v46.53,42.95 45.44,41.22 24.66,41.22 24.64,41.48 J1.1
N$2  (via drill 0.6)
  Top 0.254: IC2.53 41.88,32.61 41.88,38.89 44.17,38.89 v44.17,45.36 | 47.65,45.47 v47.83,45.47 47.83,45.36 46.79,45.36 46.79,47.12 R12.1 46.94,48.64 51.26,48.64 51.26,47.45 SW1.2
  Top 0.508: 50.78,47.59 SW1.2
  Bottom 0.254: v44.17,45.36 47.83,45.36 v47.83,45.47
N$3  (via drill 0.6)
  Top 0.178: R18.2 66.32,41.91 66.32,42.39
  Top 0.254: 66.32,42.39 v66.32,43.23 | v67.01,47.37 68.71,47.37 D2.+
  Bottom 0.254: v66.32,43.23 67.01,43.23 v67.01,47.37
N$4  (via drill 0.6)
  Top 0.178: R17.2 62.66,42.24 62.66,42.32
  Top 0.254: 62.66,42.32 v62.66,43.05 | v61.85,47.47 63.37,47.47 D1.+
  Bottom 0.254: v62.66,43.05 61.85,43.05 v61.85,47.47
N$5  (via drill 0.6)
  Top 0.178: R1.2 72.39,42.62 v72.39,42.72
  Top 0.254: 72.39,42.47 v72.39,42.72 | v72.31,47.55 74.14,47.55 D3.+
  Bottom 0.254: v72.39,42.72 72.31,42.72 v72.31,47.55
N$6
  Top 0.254: IC2.22 66.4,32.11 Y1.1
  Top 0.508: Y1.1 69.98,32.69 69.98,34.01 69.88,33.88 C14.2
N$7
  Top 0.254: Q1.3 87.96,38.53 87.96,42.98 88.85,42.98 R8.2
N$8
  Top 0.254: Y1.2 64.47,37.01 64.47,32.61 IC2.23
  Top 0.508: Y1.2 69.85,37.01 C13.2
N$9
  Top 0.254: R5.2 85.9,39.67 Q1.1
N$10
  Top 0.254: IC2.21 65.13,31.61 65.13,31.09 70.28,31.06 | 70.28,31.06 70.47,31.06 | R14.2 70.28,31.37 70.28,31.06
N$11
  Top 0.178: J10.1 10.92,36.68 R9.1
N$13
  Top 0.178: J9.1 11.4,27.15 R13.1
N$14  (via drill 0.6)
  Top 0.254: R11.1 52.15,37.95 52.15,38.86 52.78,38.86 52.78,41.3 51.94,41.3 v51.94,41.33
  Bottom 0.254: v51.94,41.33 51.49,41.33 51.49,43.99 59.54,44.02 59.64,46.74
  Bottom 0.406: 59.64,46.74 59.66,46.74 D5.+
N$15
  Top 0.508: IC7.4 76.71,10.03 C30.2
N$16
  Top 0.508: C30.1 75.34,12.45 IC7.5
N$17
  Top 0.508: IC7.1 81.43,10.95 C32.1
N$18
  Top 0.178: C32.2 83.16,13.33 83.16,13.49 83.03,13.72
  Top 0.508: IC7.3 77.98,10.03 77.98,14.6 76.96,15.57 76.96,16.89 77.57,17.4 82.19,17.4 83.03,16.61 83.03,13.72
N$19
  Top 0.508: C29.2 74.07,11.46 IC7.6
N$20
  Top 0.508: C31.1 79.15,12.75 IC7.2
N$21  (via drill 0.6)
  Top 0.254: Q2.3 51.74,43.46 51.74,43.79 51.46,43.79 v51.46,44.93
  Bottom 0.254: v51.46,44.93 57.02,44.96 57.05,46.71
  Bottom 0.406: 57.05,46.71 57.13,46.71 D5.-
N$22
  Top 0.254: IC2.60 40.41,29.11 R10.1
N$24
  Top 0.254: R15.1 17.25,21.41 D4.+
NTRST  (via drill 0.6)
  Top 0.254: J5.2 74.24,31.37 74.24,30.23 71.91,30.23 v71.91,29.87 | v54.86,27.38 56.16,27.38 56.16,23.11 IC2.4
  Bottom 0.254: v71.91,29.87 62.84,29.87 62.84,31.06 54.86,31.06 v54.86,27.38
P2_9  (via drill 0.6)
  Top 0.254: IC2.64 53.19,27.11 v53.19,30.43 | v83.97,34.85 80.82,34.85 R5.1
  Bottom 0.254: v53.19,30.43 53.19,31.78 72.8,31.7 72.8,35.08 82.12,35.13 83.97,35.13 v83.97,34.85 83.92,35.2
PWM1  (via drill 0.6)
  Top 0.254: IC6.23 49.38,11.24 v49.78,18.44 | v49.3,24.59 43.23,24.59 IC2.69
  Bottom 0.254: v49.78,18.44 49.25,18.34 v49.3,24.59
PWM2  (via drill 0.6)
  Top 0.254: IC6.15 54.58,11.24 v54.84,16.28 | v54.58,25.5 48.16,25.5 48.16,25.07 43.2,25.12 IC2.68
  Bottom 0.254: v54.84,16.28 54.79,22.48 54.1,22.48 54.1,25.5 v54.58,25.5
PWM3  (via drill 0.6)
  Top 0.254: IC5.23 28.22,15.7 28.17,16.18 28.17,19.61 v27.84,20.47 | v52.48,33.68 IC2.35
  Bottom 0.254: v27.84,20.47 27.84,34.57 27.91,34.65 51.51,34.65 v52.48,33.68
PWM4  (via drill 0.6)
  Top 0.254: IC5.15 24.51,10.5 v24.51,10.46 | v51.23,33.05 51.48,33.05 IC2.37
  Bottom 0.254: v24.51,10.46 23.5,10.39 23.5,15.87 31.62,15.85 31.62,18.69 31.57,32 31.57,32.05 31.24,32.05 31.24,34.16 51.23,34.16 v51.23,33.05
RST  (via drill 0.6)
  Top 0.254: IC2.17 60.53,29.61 | 60.53,29.62 60.53,29.61 | 60.53,28.55 v60.53,28.5 | v71.37,25.43 71.4,25.43 v71.4,16.03 | 60.53,29.61 60.53,28.55 | 63.6,30.2 63.63,28.88 62.23,28.88 62.23,28.55 60.53,28.55
  Top 0.508: R16.1 63.5,30.17 63.6,30.2
  Bottom 0.254: v60.53,28.5 66.95,28.4 66.95,26.14 71.37,26.14 v71.37,25.43 | v71.4,16.03 75.69,16.03 J5.8
RTCK  (via drill 0.6)
  Top 0.254: IC2.100 57.02,19.9 57,21.23 56.36,21.87 v56.36,22.28
  Bottom 0.254: v56.36,22.28 56.36,23.09 66.47,23.06 66.45,22.94 72.7,22.91 72.9,22.91 74.47,21.21 J5.6
RX3  (via drill 0.6)
  Top 0.254: IC2.6 60.02,24.1 60.22,24.16 60.22,24.51 60.33,24.64 62.59,24.64 63.3,23.85 v63.32,21.46
  Bottom 0.254: v63.32,21.46 67.01,21.46 CN1.2
RX_TO_TX  (via drill 0.6)
  Top 0.254: IC2.85 49.48,21.87 50.62,21.87 v50.62,21.82 | v37.9,14.68 34.06,14.71 J7.5
  Bottom 0.254: v50.62,21.82 51.26,21.82 51.26,25.65 37.85,25.65 v37.9,14.68
RXD0
  Top 0.254: IC2.99 56.46,19.86 56.46,18.82 61.7,18.82 61.7,17.12 72.85,5.97 75.03,5.97 75.36,5.64 75.36,3.81 IC7.12
RXD1  (via drill 0.6)
  Top 0.178: IC7.9 71.45,3.86 71.45,4.32 71.43,4.44
  Top 0.254: IC2.74 45.01,22.11 45.01,23.49 45.34,23.65 v55.37,23.7 | 71.43,4.44 71.43,5.51 70.94,5.99 70.74,6.17 v59.56,17.47
  Bottom 0.254: v55.37,23.7 55.45,19.81 56.67,19.81 56.67,19.74 v59.56,17.47
SER1_RX  (via drill 0.6)
  Top 0.254: IC7.13 v76.61,5.71
  Bottom 0.254: v76.61,5.71 81.18,5.71 81.18,14.6 92.35,14.6 J6.2
SER1_TX  (via drill 0.6)
  Top 0.254: IC7.14 77.85,3.78 77.85,5.87 82.42,5.87 v82.42,5.71 | v82.8,9.47 84.4,9.47 v84.4,16.94
  Bottom 0.254: v82.42,5.71 82.8,5.71 v82.8,9.47 | v84.4,16.94 92.35,16.94 J6.3
SER2_RX  (via drill 0.6)
  Top 0.508: IC7.8 71.63,9.93 71.55,9.85 71.55,8.33 73.03,6.86 78.54,6.86 78.56,7.06 87.78,7.06 87.76,7.49 v87.76,11.48
  Bottom 0.508: v87.76,11.48 88.32,11.76 J6.1
SER2_TX  (via drill 0.6)
  Top 0.508: IC7.7 72.77,10.49 72.87,8.79 73.2,8.18 85.29,8.18 v85.32,12.95
  Bottom 0.508: v85.32,12.95 85.22,13.13 J6.6
STBY  (via drill 0.6)
  Top 0.254: IC2.93 53.52,18.19 52.08,15.7 IC6.19 52.04,11.24 v52.15,9.4 | v38.56,9.96 35.59,9.96 35.74,9.88 35.51,9.96 v35.51,10.06 | v28.91,12.8 28.63,13.06 26.61,13.06 IC5.19 26.61,13.13
  Bottom 0.254: v52.15,9.4 38.53,9.37 v38.56,9.96 | v35.51,10.06 35.31,10.06 35.31,9.45 28.91,9.55 v28.91,12.8
T_RTCK
  Top 0.254: IC2.57 29.92,30.61 29.92,38.84 37.36,38.84 37.36,42.27 J1.6
  Top 0.508: J2.6 37.36,45.54 37.36,42.27
T_SRST
  Top 0.254: IC2.56 30.86,31.11 30.84,37.92 39.22,37.92 39.24,39.75 42.44,39.75 J1.8
  Top 0.508: J2.8 42.44,45.54 J1.8
T_SWDCLK  (via drill 0.6)
  Top 0.254: IC2.62 45.52,28.11 v45.52,29.46 | v36.93,29.77 29.36,29.92 29.31,39.42 34.8,39.47 J1.5
  Top 0.508: J1.5 34.87,42.85 J2.5
  Bottom 0.254: v45.52,29.46 44.81,29.46 | 44.4,29.46 44.81,29.46 | 44.81,29.46 37.29,29.49 v36.93,29.77
T_SWDIO  (via drill 0.6)
  Top 0.254: IC2.61 41.68,28.61 41.68,27.91 40.41,27.91 R10.2 39.17,27.76 39.17,27.79 35.48,27.79 35.43,28.73 28.27,28.73 28.27,41 28.5,41 v28.5,44.25
  Top 0.508: J2.4 32.28,45.54 J1.4
  Bottom 0.254: v28.5,44.25 32.33,44.25 J1.4
T_SWO
  Top 0.254: J2.7 39.98,45.54 39.98,46.84 45.48,46.84 IC2.49
  Top 0.508: J1.7 39.95,42.85 J2.7
T_TDI
  Top 0.254: IC2.58 43.31,30.11 43.31,30.1 38.15,30.05 38.15,28.57 36.04,28.57 36.04,29.21 35.94,29.21 28.85,29.16 28.8,40 29.79,40 J1.3
  Top 0.508: J2.3 30.56,45.54 30.56,45.14 30.53,45.14 30.53,42.77 29.74,42.77 J1.3
T_TRST
  Top 0.254: IC2.63 42.11,27.61 42.11,27 35,27.03 35,28.22 27.69,28.22 27.69,34.65 27.2,34.65 J1.2
  Top 0.508: J2.2 26.42,45.54 26.42,42.72 27.2,42.72 J1.2
TCK  (via drill 0.6)
  Top 0.254: v60.99,23.85 60.97,23.61 IC2.5
  Bottom 0.254: J5.5 75.31,24.13 69.19,24.13 69.19,25.3 66.57,25.3 66.37,25.15 66.32,23.85 66.04,23.57 60.96,23.6 60.96,23.82 v60.99,23.85
TDI  (via drill 0.6)
  Top 0.254: IC2.2 58.77,22.1 61.49,22.07 v61.49,22.25 | J5.3 74.27,27.36 69.95,27.36 69.95,26.8 69.95,22.73 65.46,22.73 v65.46,22.3
  Bottom 0.254: v61.49,22.25 v65.46,22.3
TDO  (via drill 0.6)
  Top 0.254: IC2.1 58.73,21.59 62.15,21.44 62.36,21.26 v62.36,20.29
  Bottom 0.254: v62.36,20.29 72.85,20.29 74.47,18.67 J5.7
TMS  (via drill 0.6)
  Top 0.254: J5.4 70.51,26.29 70.51,17.86 64.64,17.83 v64.49,18.01 | v59.87,20.47 57.48,20.65 57.43,22.61 58.7,22.61 IC2.3
  Bottom 0.254: v64.49,18.01 61.95,19.05 59.77,20.47 59.79,20.62 v59.87,20.47
TX3  (via drill 0.6)
  Top 0.254: IC2.7 57.86,24.63 v57.02,24.03 | v65.41,24.36 67.54,24.36 CN1.3
  Bottom 0.254: v57.02,24.03 59.44,24.16 59.44,25.09 63.75,25.09 63.75,24.33 v65.41,24.36
TX_TO_RX  (via drill 0.6)
  Top 0.254: v48.26,21.95 47.98,21.95 IC2.82
  Bottom 0.254: J7.1 41.55,16 41.55,19.66 40.59,19.66 40.59,22.58 44.83,22.58 44.83,20.14 48.26,20.14 v48.26,21.95
TXD0
  Top 0.254: IC2.98 56.01,19.86 56.01,18.39 60.58,18.39 60.66,17.78 60.66,17.25 71.3,6.63 71.58,6.4 72.21,5.77 72.21,5.38 74.07,5.38 IC7.11
TXD1  (via drill 0.6)
  Top 0.254: IC7.10 72.8,2.21 72.59,2.01 70.13,2.01 69.95,2.18 69.95,5.61 69.9,5.66 63.37,12.29 59.16,11.63 v58.78,11.53 | v41.68,21.39 43.01,21.39 IC2.75
  Bottom 0.254: v58.78,11.53 56.97,11.91 56.92,11.91 47.09,11.89 47.07,12.55 44.22,12.55 43.23,13.54 43.23,19.84 v41.68,21.39
VCC  (via drill 0.6)  (1 unrouted)
  Top 0.178: C6.1 21.97,32.33
  Top 0.254: 73.18,31.47 73.2,31.37 | 73.2,31.37 v73.2,35.86 | R14.1 73.2,31.37 | R11.2 52.96,37.97 v52.96,36.6
  Top 0.406: IC1.2 21.97,32.33 24.05,32.33 C8.1 | IC4.2 24.18,26.24 C7.1
  Top 0.508: J3.1 90.27,36.22 C15.2 90.25,34.11 90.25,25.15 88.72,25.15 IC3.3 | IC3.3 88.7,6.35 84.02,6.35 84.05,3.61 82.35,3.61 | 82.35,3.61 C33.2 | 82.35,3.61 80.42,3.61 IC7.16 | IC3.3 90.14,25.65 v90.14,23.82 | v26.34,27.69 24.18,27.69 C7.1 | C8.1 v26.24,32.21 | 16,4.67 14.81,4.67 14.73,0.79 9.42,0.79 9.42,9.27 9.4,9.3 9.37,20.12 16.08,20.12 16.08,23.47 17.09,23.47 17.09,26.24 IC4.2
  Bottom 0.254: v52.96,36.6 52.99,36.47 52.99,35.84
  Bottom 0.508: v90.14,23.82 88.72,23.82 88.72,35.81 v73.2,35.86 52.99,35.84 26.64,35.81 26.24,35.64 v26.24,32.21 v26.34,27.69
VDD  (via drill 0.6)
  Top 0.178: 65.63,3.96 65.56,3.96 | 65.63,3.96 IR.2 | 65.63,3.96 65.76,3.73 | v15.65,18.21 10.29,18.19 10.36,6.83 12.27,6.88 12.27,2.03 13.49,2.03 J8.10
  Top 0.254: IC2.96 54.99,17.22 55.68,17.17 55.68,15.42 57.28,15.44 57.28,15.52 | C25.1 48.34,15.8 48.34,18.03 48.98,18.03 IC2.84 | IC2.71 39.24,23.61 C19.2 | v48.49,38.35 48.98,38.35 IC2.42 | IC2.28 56.01,35.36 56.01,39.24 56.92,39.24 C2.2 58.19,39.06 58.17,39.09 58.52,39.09 | 60.22,40.36 C3.2 60.22,39.09 58.52,39.09 | IC2.19 61.37,30.61 | 61.37,30.61 61.76,30.61 61.76,30.33 | J5.1 J5.16 | 58.52,39.09 v58.52,38.35 | IC2.12 60.53,27.1 60.53,27.66 62.1,27.66 63.96,27.69 63.3,27.81 | IC2.10 57.51,26.11 57.51,27.1 IC2.12 | IC2.12 | C12.2 66.83,28.6 v68.4,28.6 | IC5.20 29.97,13.75 29.97,12.32 32.54,12.32 | 32.74,12.06 36.64,12.32 36.64,12.49 | IC2.54 41.45,32.11 41.45,33.78 40.28,33.78 C10.1 | R12.2 48.84,47.12 48.84,42.19 48.54,42.19 C1.2 | 61.37,30.23 61.37,30.61 | 61.95,30.25 61.95,31.14 64.62,31.17 64.62,28.42 | v20.5,21.59 18.95,21.59 R15.2
  Top 0.406: 61.44,1 61.44,9.07 C27.2 58.62,9.04 57.56,9.04 57.56,5.54 v58.27,5.54 | IC6.20 51.41,11.24 51.31,9.98 50.44,9.98 v50.44,8.56
  Top 0.508: C21.2 86.33,18.67 C20.2 | C20.2 86.44,22.45 IC3.2 | IC3.2 IC3.TER 86.59,32 | 86.59,32 86.49,16.71 v86.49,8.89 | v95.83,8.94 97.23,8.92 97.21,1.04 65.76,0.96 | 65.76,0.96 61.44,1 37.47,0.96 37.34,1.37 v37.31,2.26 | v37.29,11.81 36.68,11.61 | J7.6 36.64,12.49 36.68,11.61 | 36.68,11.61 41.76,11.61 J7.8 | 65.76,3.73 65.76,0.96 | 63.23,27.76 63.3,27.81 C11.2 64.62,28.42 68.4,28.42 v68.4,28.6 | C26.1 57.28,15.52 v58.45,15.52 58.45,14.27 v58.34,14.27 | v82.73,33.88 85.9,33.88 | 86.59,32 86.59,33.88 85.9,33.88 | 85.9,33.88 Q1.2 | 48.72,40.84 C1.2 48.49,40.84 v48.49,38.35 | v75.82,38.35 75.69,38.35 J5.1 | C25.1 48.39,15.8 v48.39,14.27 | C28.2 65.56,7.01 65.56,3.96 65.56,3.4 | C19.2 39.24,22.89 C18.2 26.64,22.89 26.64,20.57 25.83,20.57 v25.83,20.47 25.83,20.78 | C9.1 35.38,34.8 39.7,34.8 39.7,33.76 C10.1 40.21,33.76 v40.21,38.66 | C20.2 86.44,22.55 IC3.2 | C22.2 32.79,11.2 32.74,11.2 32.74,12.06 | 32.54,12.32 32.74,12.06 | 32.74,12.06 35.33,12.06 v35.33,11.84 | v35.36,23.42 35.33,23.42 35.33,22.94 | 61.95,30.25 61.76,30.23 | R16.2 61.72,30.23 61.76,30.23 | 61.76,30.23 61.76,30.33
  Bottom 0.178: IR.2 65.58,3.73 | v15.65,18.21 20.5,20.85
  Bottom 0.254: J5.1 74.09,33.91 74.09,33.27 | 22.78,20.47 20.5,20.47 20.5,20.85 v20.5,21.59
  Bottom 0.406: v50.44,8.56 58.27,8.56 v58.27,5.54
  Bottom 0.508: v86.49,8.89 94.29,8.94 v95.83,8.94 | v37.31,2.26 v37.29,11.81 | v58.45,15.52 61.49,15.52 61.49,10.44 62.94,10.44 62.94,8.61 65.58,8.58 65.58,3.73 | v68.4,28.6 73.89,28.6 73.89,28.7 74.09,28.7 74.09,33.27 74.09,34.09 82.73,34.09 v82.73,33.88 | v75.82,38.35 v58.52,38.35 v48.49,38.35 48.49,38.66 v40.21,38.66 22.78,38.66 22.78,20.47 v25.83,20.47 | v48.39,14.27 v58.34,14.27 | v35.33,11.84 v35.36,23.42

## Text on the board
Bottom: TWI 9/15
tNames: Target | JTAG | CAN | Serial | ESP-01 | MOTOR
bNames: This is open hardware, CAD Files and firmware source / https://github.com/TWilmer/targetboard | Features: / + simulate trafic light / + usb to serial / + usb to CAN / + usb to JTAG / + 4 motor control for robot kit / + Wifi module support / / This board is intended for Personal/Hobby use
